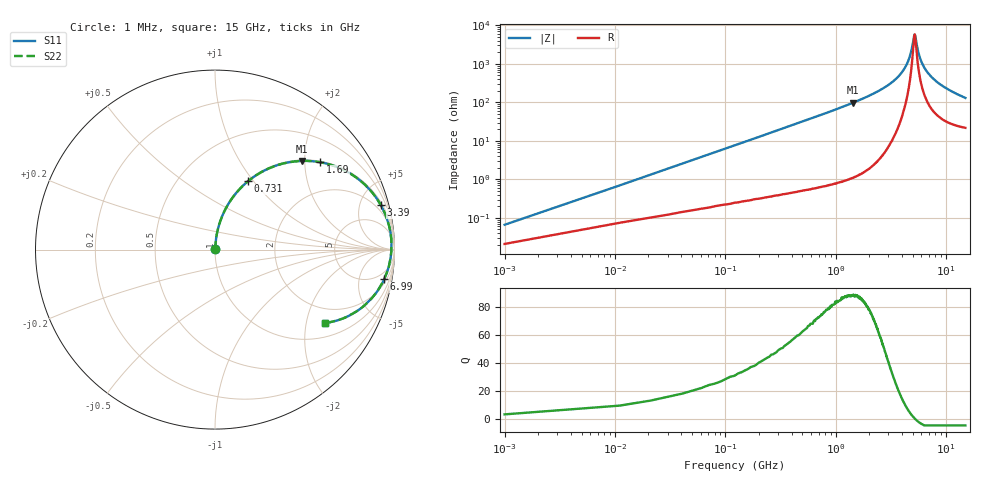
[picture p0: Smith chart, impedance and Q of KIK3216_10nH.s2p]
!version-2
!date-01.2022
!Series
# MHz S RI R 50
!Freq ReS11 ImS11 ReS21 ImS21 ReS12 ImS12 ReS22 ImS22
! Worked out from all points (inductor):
!   1501 points, 1 MHz to 15 GHz, reference 50 ohm
!   read as one part in series: L = 10 nH near 71 MHz
!   highest Q = 88.5 at 1.43 GHz (marker M1), where L = 10.8 nH
!   self-resonance near 5.211 GHz
!   S11 on the Smith chart (normalised r, x): 1 MHz: 1.00, +0.00; 731 MHz: 1.01, +0.94; 1.69 GHz: 1.03, +2.38; 3.39 GHz: 1.26, +7.39; 6.99 GHz: 3, -11; 15 GHz: 1.44, -2.57
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1  0.000222 0.000628  0.9998 -0.000628  0.9998 -0.000628  0.000222 0.000628
81  0.00457 0.0506  0.9954 -0.0506  0.9954 -0.0506  0.00457 0.0506
111  0.00715 0.0691  0.9929 -0.0691  0.9929 -0.0691  0.00715 0.0691
161  0.0129 0.0997  0.9871 -0.0997  0.9871 -0.0997  0.0129 0.0997
371  0.0557 0.2203  0.9443 -0.2203  0.9443 -0.2203  0.0557 0.2203
731  0.1833 0.3802  0.8167 -0.3802  0.8167 -0.3802  0.1833 0.3802
1430  0.4863 0.4942  0.5137 -0.4942  0.5137 -0.4942  0.4863 0.4942
1690  0.5843 0.4871  0.4157 -0.4871  0.4157 -0.4871  0.5843 0.4871
2510  0.8046 0.3882  0.1954 -0.3882  0.1954 -0.3882  0.8046 0.3882
3390  0.9243 0.2475  0.0757 -0.2475  0.0757 -0.2475  0.9243 0.2475
4430  0.9775 0.0958  0.0225 -0.0958  0.0225 -0.0958  0.9775 0.0958
4760  0.9824 0.0534  0.0176 -0.0534  0.0176 -0.0534  0.9824 0.0534
5010  0.9835 0.0232  0.0165 -0.0232  0.0165 -0.0232  0.9835 0.0232
5140  0.9833 0.00804  0.0167 -0.00804  0.0167 -0.00804  0.9833 0.00804
5230  0.9829 -0.00218  0.0171 0.00218  0.0171 0.00218  0.9829 -0.00218
5580  0.9793 -0.0401  0.0207 0.0401  0.0207 0.0401  0.9793 -0.0401
5890  0.9739 -0.0713  0.0261 0.0713  0.0261 0.0713  0.9739 -0.0713
6990  0.9424 -0.1658  0.0576 0.1658  0.0576 0.1658  0.9424 -0.1658
7510  0.9231 -0.2027  0.077 0.2027  0.077 0.2027  0.9231 -0.2027
10010  0.8145 -0.3259  0.1855 0.3259  0.1855 0.3259  0.8145 -0.3259
12510  0.7058 -0.3863  0.2942 0.3863  0.2942 0.3863  0.7058 -0.3863
15000  0.6116 -0.4098  0.3884 0.4098  0.3884 0.4098  0.6116 -0.4098
